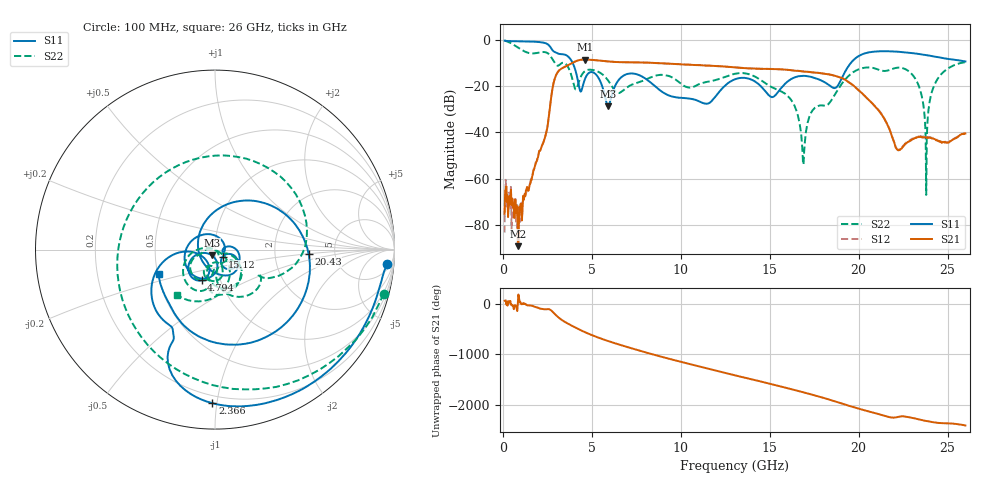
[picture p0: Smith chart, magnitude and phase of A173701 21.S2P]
!  2-Port S-parameters saved by WinCal
! VAR MeasName=S-Parameters (CALIBRATED_DATA) read from VNA (N5245A)
! VAR MeasDate=2017-6-7 10:29:46
! VAR NAME=A173701 21
! VAR FILENAME=A173701 21.S2P
! VAR DATE=2017-6-7 10:29:46
! VAR PHYS_PORTS=1,2
# Hz S DB R 50
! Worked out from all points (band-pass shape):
!   801 points, 100 MHz to 26 GHz, reference 50 ohm
!   highest |S21| = -8.50 dB at 4.633 GHz (marker M1); lowest = -89.2 dB at 877 MHz (marker M2)
!   |S21| within 3 dB of the highest: 3.531 GHz to 12.42 GHz (8.888 GHz wide, 111 % of centre)
!   lowest |S11| = -28.8 dB at 5.928 GHz (marker M3), VSWR 1.08, Z = 48.2 - j3.1 ohm
!   |S11| at or under -10 dB: 3.928 GHz to 19.56 GHz (15.63 GHz wide, 133 % of centre)
!   |S22| runs from -67.0 to -0.2 dB; largest |S21 - S12| = 0.0038
!   S11 on the Smith chart (normalised r, x): 100 MHz: 9, -20; 2.366 GHz: 0.15, -0.97; 4.794 GHz: 0.82, -0.29; 15.12 GHz: 1.09, -0.09; 20.43 GHz: 3.17, -0.21; 26 GHz: 0.51, -0.15
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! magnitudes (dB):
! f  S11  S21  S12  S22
! 100 MHz  -0.3  -75.2  -83.3  -0.2
! 877 MHz  -0.6  -89.2  -79.8  -3.4
! 2.366 GHz  -1.4  -42.2  -42.2  -5.3
! 3.014 GHz  -5.6  -14.9  -14.9  -10.8
! 4.438 GHz  -21.5  -8.6  -8.6  -15.1
! 4.633 GHz  -16.6  -8.5  -8.5  -13.4
! 4.794 GHz  -14.6  -8.6  -8.5  -12.9
! 5.928 GHz  -28.8  -9.3  -9.3  -17.7
! 6.996 GHz  -14.7  -9.7  -9.7  -20.5
! 8.744 GHz  -21.2  -10.0  -10.1  -15.2
! 11.46 GHz  -27.6  -11.1  -11.1  -18.2
! 13.05 GHz  -17.0  -11.9  -11.9  -14.6
! 15.12 GHz  -24.8  -12.6  -12.6  -20.5
! 16.32 GHz  -16.5  -13.2  -13.1  -27.3
! 16.87 GHz  -15.6  -13.7  -13.6  -52.8
! 17.39 GHz  -16.1  -14.1  -14.0  -30.7
! 20.43 GHz  -5.6  -25.0  -24.9  -11.9
! 21.69 GHz  -4.9  -38.0  -37.9  -13.1
! 23.15 GHz  -5.9  -42.5  -42.3  -16.4
! 23.8 GHz  -6.6  -42.3  -41.9  -67.0
! 24.41 GHz  -7.4  -43.6  -43.1  -17.2
! 26 GHz  -9.3  -40.5  -40.4  -9.7
